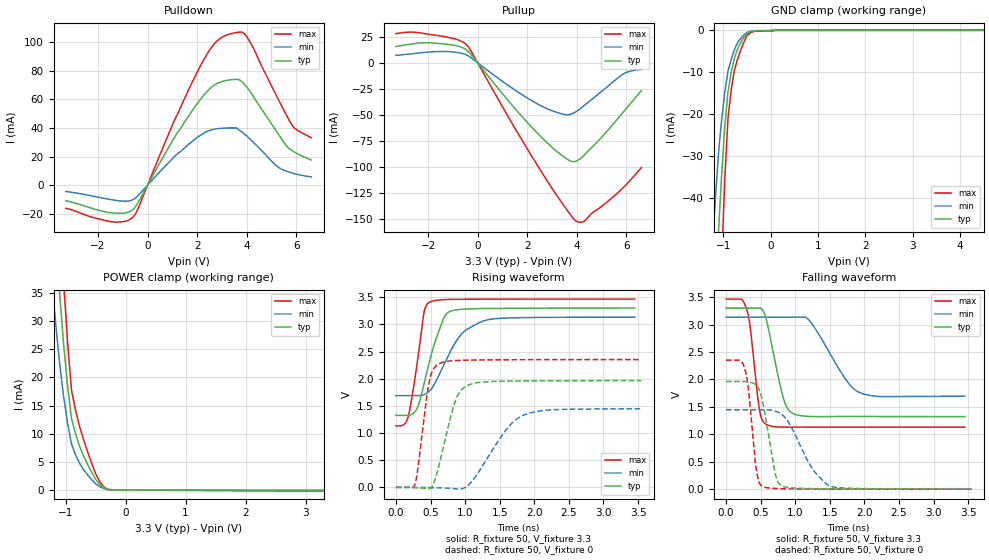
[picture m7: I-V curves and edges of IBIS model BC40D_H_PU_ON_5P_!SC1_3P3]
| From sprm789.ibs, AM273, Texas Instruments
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|   Model Cell BC40D_H_PU_ON_5P_!SC1_3P3
|BC40D_H_PU_ON_5P_!SC1_3P3
[Model]   BC40D_H_PU_ON_5P_!SC1_3P3
Model_type   I/O
Polarity   Non-Inverting
Enable   Active-Low
Vinl =  0.8V
Vinh =  2V
Cref =  15pF
Rref =  100.0000M
Vref =  0V
Vmeas =  1.65
C_comp   2.157014p   1.964007p   2.198404p
|[Input load] weak_pu_on
|[Output drive] fast
|[supplytol] 5
|[temp] ind
[Model Spec]
Vinl   0.8V   0.8V   0.8V
Vinh   2V   2V   2V
[Temperature Range]   25   125   -40
[Voltage Range]   3.3   3.135   3.465
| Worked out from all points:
|   slope of the pulldown table from 0 to 0.495 V, typ, clamps not added: 31.8 ohm
|   slope of the pullup table from 0 to 0.495 V, typ, clamps not added: 33.3 ohm
|   GND clamp passes 1 mA (typ) near -0.52 V on its own axis
|   POWER clamp passes 1 mA (typ) near -0.43 V on its own axis
|   rising waveform, R_fixture 50, V_fixture 3.3: 20-80 % time 258ps typ, 377ps min, 156ps max; typ from 1.32 V to 3.3 V
|   rising waveform, R_fixture 50, V_fixture 0: 20-80 % time 233ps typ, 458ps min, 142ps max; typ from 0 V to 1.97 V
|   falling waveform, R_fixture 50, V_fixture 3.3: 20-80 % time 199ps typ, 410ps min, 121ps max; typ from 3.3 V to 1.32 V
|   falling waveform, R_fixture 50, V_fixture 0: 20-80 % time 162ps typ, 365ps min, 108ps max; typ from 1.96 V to 0.003 V
| Nom Voltages:
|   VDD=1.1, VDDS=3.3, VDDS18=1.8, ESD_BIASFET=0, VSS=0, VSSS=0
| Min Voltages:
|   VDD=1.045, VDDS=3.135, VDDS18=1.71, ESD_BIASFET=0, VSS=0, VSSS=0
| Max Voltages:
|   VDD=1.16, VDDS=3.465, VDDS18=1.89, ESD_BIASFET=0, VSS=0, VSSS=0
[POWER_clamp]
|   voltage   I(typ)   I(min)   I(max)
-3.3V     446.9mA    437.1mA    604mA
-1.233V   56.55mA    37.5mA     80.28mA
-1.167V   45.63mA    29.89mA    65.07mA
-1.1V     35.1mA     22.65mA    50.26mA
-1.033V   26.08mA    16.75mA    37.2mA
-966.7mV  18.62mA    11.92mA    26.34mA
-900mV    12.7mA     8.144mA    17.7mA
-833.3mV  10mA       6.261mA    14.22mA
-766.7mV  7.795mA    4.75mA     11.31mA
-566.7mV  3.199mA    1.871mA    4.824mA
-366.7mV  433.5uA    268.9uA    617.1uA
3.3V      -100.3uA   -54.66uA   -173.1uA
[Pulldown]
|   voltage   I(typ)   I(min)   I(max)
-3.3V     -10.92mA   -4.469mA   -16.24mA
-1.4V     -19.52mA   -10.37mA   -25.81mA
-600mV    -17.22mA   -10.34mA   -22.6mA
-400mV    -12.67mA   -7.623mA   -17.05mA
1.2V      36.7mA     21.92mA    49.35mA
2.1V      59.3mA     34.49mA    82.4mA
2.7V      70.09mA    39.15mA    99.03mA
3.3V      73.56mA    39.95mA    105.7mA
3.9V      70.66mA    35.84mA    106mA
5.2V      37.64mA    13.39mA    62.46mA
5.8V      24.43mA    8.578mA    42.66mA
6.6V      17.6mA     5.765mA    33.17mA
[Pullup]
|   voltage   I(typ)   I(min)   I(max)
-3.3V     15.77mA    7.22mA     28.03mA
-2.7V     18.05mA    8.673mA    29.54mA
-1.9V     19.23mA    10.53mA    27.2mA
-900mV    16.69mA    10.25mA    22.94mA
-400mV    11.53mA    6.969mA    16.15mA
1.4V      -40.96mA   -24.37mA   -58.54mA
2.6V      -72.01mA   -41.71mA   -105.6mA
3.6V      -92.16mA   -49.74mA   -141mA
4V        -93.89mA   -46.2mA    -152.2mA
4.3V      -88.33mA   -40.72mA   -151.7mA
5.9V      -46.29mA   -10.2mA    -118.8mA
6.6V      -26.71mA   -6.269mA   -100.4mA
[GND_clamp]
|   voltage   I(typ)   I(min)   I(max)
-3.3V     -787.2mA   -627.7mA   -1.235A
-1.233V   -85.67mA   -52.14mA   -138.8mA
-1.167V   -66.48mA   -40.37mA   -107.8mA
-1.1V     -48.26mA   -29.38mA   -78.01mA
-1.033V   -34.3mA    -21.2mA    -54.61mA
-966.7mV  -23.1mA    -14.68mA   -35.59mA
-900mV    -14.66mA   -9.807mA   -20.94mA
-833.3mV  -10.12mA   -6.96mA    -14.29mA
-700mV    -4.501mA   -2.971mA   -6.963mA
-500mV    -717.7uA   -493.4uA   -1.261mA
100mV     0A         0A         0A
6.6V      0A         0A         0A
[Ramp]
| variable   typ   min   max
dV/dt_f  1.1950009/0.20080853n 0.88975764/0.42406791n  1.4061698/0.12174193n
dV/dt_r  1.1920104/0.23568046n 0.88882206/0.46966013n  1.4196578/0.14317133n
R_load = 50
[Rising Waveform]
R_fixture = 50
V_fixture = 3.3
V_fixture_min = 3.135
V_fixture_max = 3.465
|   time   V(typ)   V(min)   V(max)
0s        1.324V     1.688V     1.132V
177.2ps   1.325V     1.688V     1.301V
303.7ps   1.447V     1.688V     2.256V
400.3ps   1.875V     1.703V     3.18V
485.8ps   2.322V     1.773V     3.407V
661.9ps   3.024V     2.171V     3.452V
735.5ps   3.198V     2.369V     3.457V
959.3ps   3.277V     2.836V     3.461V
1.253ns   3.291V     3.057V     3.463V
3.453ns   3.299V     3.131V     3.465V
[Rising Waveform]
R_fixture = 50
V_fixture = 0
V_fixture_min = 0
V_fixture_max = 0
|   time   V(typ)   V(min)   V(max)
0s        0V         0V         3.507mV
274.9ps   -4.733mV   0V         55.55mV
480.1ps   -20.97mV   -3.534mV   1.936V
543.7ps   69.38mV    -5.301mV   2.181V
622.4ps   404.7mV    -7.595mV   2.273V
859ps     1.592V     -25.75mV   2.334V
1.054ns   1.886V     51.53mV    2.342V
1.594ns   1.956V     1.061V     2.348V
1.846ns   1.959V     1.33V      2.35V
3.547ns   1.965V     1.444V     2.352V
[Falling Waveform]
R_fixture = 50
V_fixture = 3.3
V_fixture_min = 3.135
V_fixture_max = 3.465
|   time   V(typ)   V(min)   V(max)
0s        3.3V       3.134V     3.464V
301ps     3.3V       3.134V     3.266V
351.3ps   3.3V       3.134V     2.93V
482.7ps   3.3V       3.134V     1.45V
582.8ps   3.088V     3.134V     1.181V
827.6ps   1.663V     3.134V     1.132V
969.8ps   1.379V     3.134V     1.132V
1.206ns   1.326V     3.071V     1.133V
1.923ns   1.327V     1.766V     1.131V
3.453ns   1.324V     1.696V     1.131V
[Falling Waveform]
R_fixture = 50
V_fixture = 0
V_fixture_min = 0
V_fixture_max = 0
|   time   V(typ)   V(min)   V(max)
0s        1.964V     1.449V     2.351V
273.2ps   1.964V     1.449V     2.184V
322.1ps   1.961V     1.449V     1.833V
438.5ps   1.891V     1.449V     343.6mV
525.2ps   1.614V     1.449V     54.57mV
714.7ps   268.2mV    1.423V     15.15mV
817.3ps   55.88mV    1.353V     9.958mV
1.24ns    12.36mV    391.8mV    4.301mV
1.506ns   8.628mV    60.15mV    3.207mV
3.547ns   2.504mV    4.605mV    2.797mV
